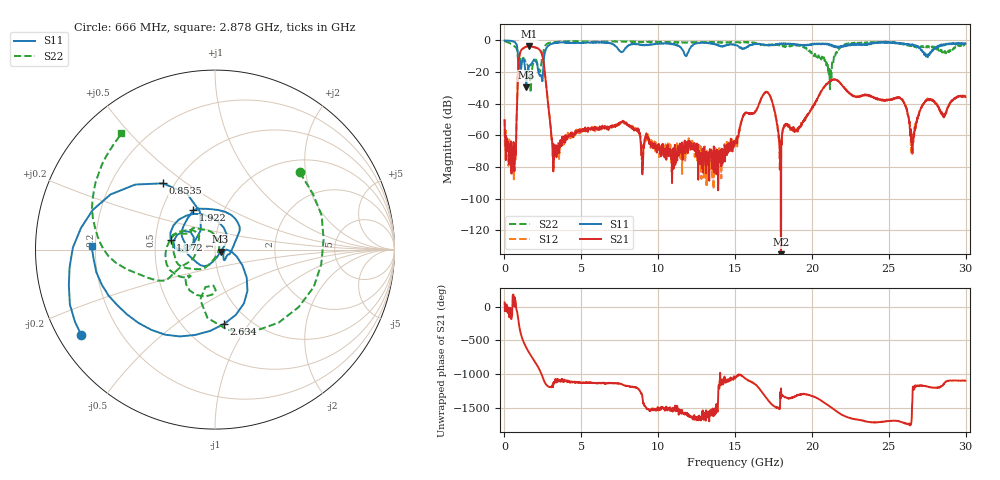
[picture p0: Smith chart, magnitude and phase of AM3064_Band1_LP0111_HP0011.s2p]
# Hz S DB R 50.0
!freq dBS11 angS11 dBS21 angS21 dBS12 angS12 dBS22 angS22
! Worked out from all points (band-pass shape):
!   1600 points, 10 MHz to 29.98 GHz, reference 50 ohm
!   highest |S21| = -3.69 dB at 1.584 GHz (marker M1); lowest = -198.7 dB at 17.99 GHz (marker M2)
!   |S21| within 3 dB of the highest: 1.061 GHz to 2.348 GHz (1.287 GHz wide, 75.5 % of centre)
!   lowest |S11| = -29.7 dB at 1.416 GHz (marker M3), VSWR 1.07, Z = 53.2 - j1.15 ohm
!   |S11| at or under -10 dB: 876.6 MHz to 2.588 GHz (1.711 GHz wide, 98.8 % of centre); 27.41237 GHz to 27.43687 GHz (24.5 MHz wide, 0.0893 % of centre); 27.51215 GHz to 27.55171 GHz (39.56 MHz wide, 0.144 % of centre)
!   |S22| runs from -32.9 to -0.3 dB; largest |S21 - S12| = 0.0086
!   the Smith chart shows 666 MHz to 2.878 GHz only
!   S11 on the Smith chart (normalised r, x): 666 MHz: 0.07, -0.29; 853.5 MHz: 0.43, +0.41; 1.172 GHz: 0.60, +0.07; 1.922 GHz: 0.72, +0.34; 2.634 GHz: 0.77, -0.77; 2.878 GHz: 0.18, +0.01
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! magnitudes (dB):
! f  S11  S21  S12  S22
! 10 MHz  -0.1  -50.7  -49.6  -0.3
! 666 MHz  -1.1  -69.5  -82.3  -3.9
! 853.5 MHz  -6.6  -27.9  -27.8  -8.3
! 1.172 GHz  -11.9  -5.4  -5.3  -11.7
! 1.416 GHz  -29.7  -3.9  -3.9  -15.4
! 1.584 GHz  -16.7  -3.7  -3.7  -18.7
! 1.922 GHz  -12.0  -4.3  -4.2  -12.9
! 2.634 GHz  -7.6  -21.1  -21.0  -3.8
! 2.878 GHz  -3.2  -43.3  -43.3  -1.6
! 3.29 GHz  -1.7  -69.4  -68.9  -1.0
! 5.015 GHz  -1.4  -56.9  -57.2  -0.6
! 10 GHz  -2.1  -66.2  -66.9  -0.9
! 15 GHz  -2.9  -64.9  -66.6  -1.3
! 17.03 GHz  -3.1  -32.5  -32.5  -3.4
! 17.99 GHz  -2.4  -198.7  -64.5  -3.4
! 19.99 GHz  -2.9  -43.0  -42.7  -8.1
! 21.42 GHz  -3.8  -24.7  -24.5  -11.2
! 25 GHz  -1.0  -37.3  -37.3  -1.3
! 25.95 GHz  -1.8  -38.6  -38.6  -2.7
! 26.53 GHz  -2.4  -71.1  -71.6  -4.3
! 27.43 GHz  -10.2  -38.0  -37.8  -3.9
! 29.98 GHz  -1.9  -35.8  -35.3  -3.0
